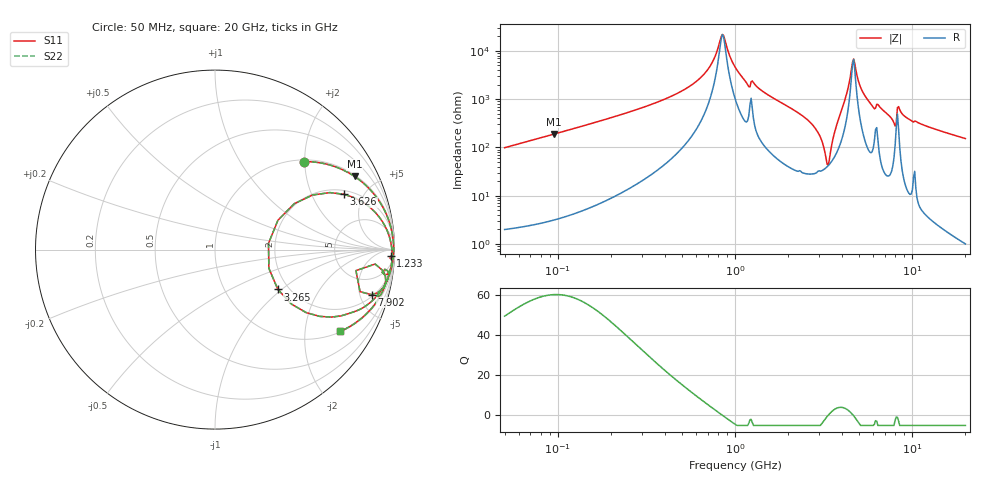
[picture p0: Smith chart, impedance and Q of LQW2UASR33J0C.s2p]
!Murata Part Number: LQW2UASR33J0C
!These Parameters are Measured in Series Mode Connection
!  o--[Z]--o
!Port1  Port2
!  o-------o
!Freq. Start=50[MHz] Stop=20[GHz], 401[Steps]
# Hz S RI R 50
!Freq.(Hz) S11(Real) S11(Imag) S21(Real) S21(Imag) S12(Real) S12(Imag) S22(Real) S22(Imag)
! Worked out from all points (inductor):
!   401 points, 50 MHz to 20 GHz, reference 50 ohm
!   read as one part in series: L = 313 nH near 51.52 MHz
!   highest Q = 60.4 at 95.21 MHz (marker M1), where L = 317 nH
!   self-resonance near 848.1 MHz
!   S11 on the Smith chart (normalised r, x): 50 MHz: 1.04, +1.97; 1.233 GHz: 22, -41; 3.265 GHz: 1.76, -0.94; 3.626 GHz: 2.23, +3.54; 7.902 GHz: 2.21, -6.33; 20 GHz: 1.02, -3.06
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5e7  0.4938 0.49  0.5062 -0.49  0.5062 -0.49  0.4938 0.49
9.521195e7  0.7782 0.4073  0.2218 -0.4073  0.2218 -0.4073  0.7782 0.4073
1.364002e8  0.8787 0.3178  0.1213 -0.3178  0.1213 -0.3178  0.8787 0.3178
3.721004e8  0.9834 0.1092  0.0166 -0.1092  0.0166 -0.1092  0.9834 0.1092
6.476653e8  0.9945 0.0336  0.0055 -0.0336  0.0055 -0.0336  0.9945 0.0336
7.411344e8  0.9953 0.017  0.00471 -0.017  0.00471 -0.017  0.9953 0.017
8.480927e8  0.9955 0.000465  0.00451 -0.000465  0.00451 -0.000465  0.9955 0.000465
1e9  0.9948 -0.0207  0.00519 0.0207  0.00519 0.0207  0.9948 -0.0207
1.23331e9  0.9792 -0.0372  0.0208 0.0372  0.0208 0.0372  0.9792 -0.0372
2.728004e9  0.8784 -0.283  0.1216 0.283  0.1216 0.283  0.8784 -0.283
3.075291e9  0.6473 -0.3761  0.3527 0.3761  0.3527 0.3761  0.6473 -0.3761
3.265178e9  0.3501 -0.2219  0.6499 0.2219  0.6499 0.2219  0.3501 -0.2219
3.415248e9  0.3504 0.163  0.6496 -0.163  0.6496 -0.163  0.3504 0.163
3.626126e9  0.7191 0.3083  0.2809 -0.3083  0.2809 -0.3083  0.7191 0.3083
3.967106e9  0.9311 0.1584  0.0689 -0.1584  0.0689 -0.1584  0.9311 0.1584
4.677679e9  0.9857 -0.00256  0.0143 0.00256  0.0143 0.00256  0.9857 -0.00256
5.598765e9  0.9802 -0.098  0.0198 0.098  0.0198 0.098  0.9802 -0.098
7.442007e9  0.9423 -0.2061  0.0577 0.2061  0.0577 0.2061  0.9423 -0.2061
7.901521e9  0.8725 -0.2512  0.1275 0.2512  0.1275 0.2512  0.8725 -0.2512
8.516016e9  0.9495 -0.1503  0.0505 0.1503  0.0505 0.1503  0.9495 -0.1503
9.892087e9  0.922 -0.2536  0.078 0.2536  0.078 0.2536  0.922 -0.2536
2e10  0.699 -0.4554  0.301 0.4554  0.301 0.4554  0.699 -0.4554
